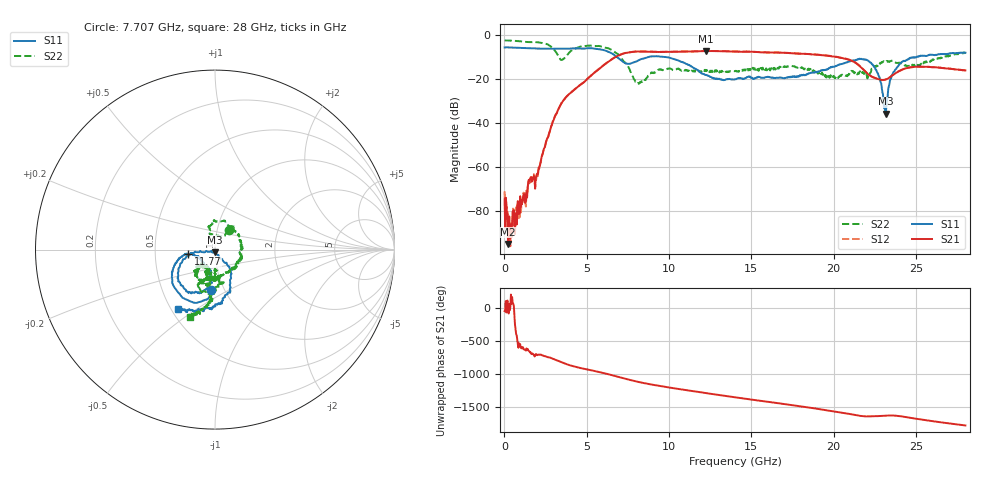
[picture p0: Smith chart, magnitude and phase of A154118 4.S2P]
!  2-Port S-parameters saved by WinCal
! VAR MeasName=S-Parameters (CALIBRATED_DATA) read from VNA (N5230A)
! VAR MeasDate=2015-9-10 14:34:45
! VAR NAME=A154118 4
! VAR FILENAME=A154118 4.S2P
! VAR DATE=2015-9-10 14:34:45
! VAR PHYS_PORTS=1,2
# Hz S DB R 50
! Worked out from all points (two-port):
!   801 points, 10 MHz to 28 GHz, reference 50 ohm
!   highest |S21| = -7.44 dB at 12.26 GHz (marker M1); lowest = -95.1 dB at 219.9 MHz (marker M2)
!   |S21| within 3 dB of the highest: 6.687 GHz to 20.37 GHz (13.68 GHz wide, 101 % of centre)
!   lowest |S11| = -36.0 dB at 23.17 GHz (marker M3), VSWR 1.03, Z = 50.1 - j1.58 ohm
!   |S11| at or under -10 dB: 6.793 GHz to 8.827 GHz (2.034 GHz wide, 26 % of centre); 9.446 GHz to 25.06 GHz (15.61 GHz wide, 90.5 % of centre); 25.07959 GHz to 25.13229 GHz (52.69 MHz wide, 0.21 % of centre)
!   |S22| runs from -22.3 to -2.7 dB; largest |S21 - S12| = 0.0076
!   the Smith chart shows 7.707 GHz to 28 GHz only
!   S11 on the Smith chart (normalised r, x): 7.707 GHz: 0.87, -0.41; 11.77 GHz: 0.74, -0.04; 28 GHz: 0.55, -0.42
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1e7  -5.84 179.6  -74.83 -42.8  -71.24 -93.5  -2.67 179.8
2.19925e8  -5.82 172.3  -95.07 -22.1  -81.54 113.0  -2.70 174.6
7.79725e8  -5.99 153.5  -77.43 -125.8  -78.87 -122.8  -2.89 160.6
1.9693e9  -6.32 113.3  -63.49 13.9  -63.37 10.9  -3.48 129.1
2.66905e9  -6.43 87.0  -46.12 -24.8  -45.95 -24.8  -4.67 91.1
3.193862e9  -6.39 65.3  -35.31 -72.3  -35.34 -72.3  -8.71 25.7
3.753662e9  -6.37 40.6  -28.30 -128.4  -28.30 -128.3  -9.83 -108.9
4.698325e9  -6.35 -4.3  -22.35 166.4  -22.33 166.5  -5.35 166.3
6.1678e9  -7.35 -75.3  -13.09 86.0  -13.01 85.9  -6.01 102.2
7.70725e9  -13.00 -95.1  -7.98 -15.1  -7.88 -15.3  -17.65 54.9
9.351662e9  -9.88 -125.9  -7.91 -98.7  -7.82 -99.0  -15.98 94.1
1.17658e10  -16.42 -171.0  -7.58 168.1  -7.54 167.3  -16.55 -0.2
1.225562e10  -18.36 -165.0  -7.44 149.7  -7.41 148.9  -16.61 -20.8
1.4005e10  -20.31 -135.9  -7.73 86.4  -7.71 85.8  -16.63 -76.4
1.645412e10  -19.78 -123.9  -8.16 2.5  -8.14 2.1  -15.91 -103.5
1.869332e10  -17.21 -100.5  -8.98 -77.0  -8.97 -77.4  -15.85 -129.0
2.198215e10  -11.43 -139.5  -17.24 155.3  -17.18 154.5  -18.36 -90.7
2.264691e10  -17.30 -171.3  -20.04 159.6  -20.11 158.7  -14.34 -79.5
2.317172e10  -35.99 -84.1  -20.35 168.4  -20.29 168.0  -12.26 -96.5
2.334666e10  -23.57 -52.5  -19.69 170.5  -19.63 170.2  -12.34 -102.0
2.460621e10  -10.90 -81.5  -15.00 136.1  -14.92 134.9  -14.29 -111.6
2.8e10  -8.25 -121.8  -16.26 17.9  -16.26 17.2  -7.93 -109.9
